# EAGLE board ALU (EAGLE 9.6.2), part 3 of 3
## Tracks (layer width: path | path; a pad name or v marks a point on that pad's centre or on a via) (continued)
N/IN/N2  (via drill 0.35) (continued)
  Top 0.152: IC70.9 99.06,26.09 99.32,26.35 v99.54,26.35 | IC63.10 127,41.28 v127.48,40.8
  Route3 0.152: v99.54,26.35 103.5,26.35 108.74,31.59 109.7,31.59 118.75,40.64 120.65,40.64 122.56,42.55 125.73,42.55 v127.48,40.8
  Bottom 0.152: 101.44,24.45 v99.54,26.35
N/IN/N3  (via drill 0.35)
  Top 0.152: v99.06,15.24 IC70.6 | v125.73,40.96 IC63.11
  Route3 0.152: v125.73,40.96 125.73,39.69 113.67,27.62 112.08,27.62 99.69,15.24 v99.06,15.24
STA  (via drill 0.35)
  Top 0.152: v109.22,46.99 IC67.13 | v139.7,47.47 IC56.13
  Route14 0.152: v139.7,47.47 139.38,47.15 114.14,47.15 113.19,46.2 110.01,46.2 v109.22,46.99
  Route15 0.152: v109.22,46.99 78.74,16.51 W.1
SUA  (via drill 0.35)
  Top 0.152: v113.03,40.64 IC66.10 | v115.41,56.2 111.44,56.2 110.49,57.15 IC68.12 | v139.7,67.31 IC58.13
  Route3 0.152: v139.7,67.31 135.57,63.18 122.4,63.18 v115.41,56.2 115.41,52.23 115.09,51.91 115.09,48.58 117,46.67 117,43.82 113.82,40.64 v113.03,40.64
SUB/IN/Z-/N0/0  (via drill 0.35)
  Top 0.152: v45.72,62.71 48.26,62.71 IC21.1 | v57.15,62.87 62.23,62.87 IC22.1 | v69.22,76.2 IC26.10
  Route2 0.152: v57.15,62.87 56.99,62.71 v45.72,62.71
  Route3 0.152: v69.22,76.2 65.88,72.87 65.88,70.96 65.41,70.48 63.5,70.48 57.15,64.14 v57.15,62.87
SUB/IN/Z-/N1/0
  Top 0.152: IC21.8 55.88,71.12 60.64,75.88 66.36,75.88 67.94,74.3 IC26.6 67.94,72.39 68.58,71.75 69.22,71.75 69.85,71.12 IC22.8
SUB/IN/Z-/N2/0  (via drill 0.35)
  Top 0.152: IC25.1 7.62,61.59 8.26,60.96 v8.89,60.96 | v64.14,74.93 64.77,74.93 65.41,74.3 IC26.4 | v19.37,62.71 19.37,62.87 19.47,62.97 IC24.1
  Route3 0.152: v64.14,74.93 57.78,68.58 35.56,68.58 34.77,69.37 32.54,69.37 31.27,70.64 29.53,70.64 21.59,62.71 v19.37,62.71
  Route14 0.152: v19.37,62.71 17.78,62.71 14.92,59.85 10,59.85 v8.89,60.96
SUB/IN/Z-/N3/0  (via drill 0.35)
  Top 0.152: IC25.8 15.24,70.48 16.51,71.75 26.67,71.75 27.94,70.48 27.94,69.22 | v59.69,73.66 60.96,74.93 62.55,74.93 62.87,74.61 IC26.2 | 27.94,69.22 v29.84,67.31 | 27.94,69.22 IC24.8
  Route2 0.152: v59.69,73.66 46.99,73.66 40.64,67.31 v29.84,67.31
SUB/OUT/N0  (via drill 0.35)
  Top 0.152: IC48.13 8.89,80.64 11.43,83.19 19.05,83.19 31.75,70.48 v31.75,66.04 | v31.75,51.44 32.38,50.8 36.2,50.8 36.83,51.44 IC18.3
  Bottom 0.152: v31.75,51.44 31.75,60.33 v31.75,66.04
SUB/OUT/N1  (via drill 0.35)
  Top 0.152: IC18.4 38.1,51.12 37.15,50.16 31.43,50.16 30.48,51.12 v30.48,54.61 | IC48.9 13.97,78.11 14.61,77.47 24.13,77.47 31.11,70.48 31.11,66.83 30.48,66.2 v30.48,64.77
  Bottom 0.152: v30.48,64.77 v30.48,54.61
SUB/OUT/N2  (via drill 0.35)
  Top 0.152: v29.53,69.37 29.53,70.8 25.4,74.93 14.61,74.93 13.97,74.3 IC48.6 | v36.83,60.64 39.05,60.64 39.37,60.33 IC18.10
  Route3 0.152: v29.53,69.37 36.83,62.07 v36.83,60.64
SUB/OUT/N3  (via drill 0.35)
  Top 0.152: v8.89,74.93 IC48.2 | IC18.11 v38.1,57.47
  Route15 0.152: v38.1,57.47 37.62,57.94 33.5,57.94 31.91,56.36 27.46,56.36 v8.89,74.93
SUB/OUT/Z-/N0  (via drill 0.35)
  Top 0.152: IC23.3 36.83,61.59 37.31,61.12 43.66,61.12 v48.26,56.52 49.53,55.25 IC16.2 | IC17.2 63.5,52.07 v62.23,50.8
  Route14 0.152: v48.26,56.52 48.58,56.2 54.61,56.2 58.98,51.83 61.2,51.83 v62.23,50.8
SUB/OUT/Z-/N1  (via drill 0.35)
  Top 0.152: IC23.4 38.1,61.91 38.42,61.59 46.67,61.59 v47.31,60.96 | v53.98,57.15 54.61,57.79 IC16.9 | v68.58,57.47 IC17.9
  Route2 0.152: v47.31,60.96 49.53,60.96 53.34,57.15 v53.98,57.15 54.45,57.63 63.34,57.63 65.09,55.88 66.99,55.88 v68.58,57.47
SUB/OUT/Z-/N2  (via drill 0.35)
  Top 0.152: IC19.2 21.59,54.61 20,56.2 17.46,56.2 16.35,55.09 9.68,55.09 v8.89,54.29 IC20.2 | IC23.10 39.37,71.12 37.47,73.03 v36.2,73.03
  Route2 0.152: v36.2,73.03 10.16,73.03 7.62,70.48 7.62,55.56 v8.89,54.29
SUB/OUT/Z-/N3  (via drill 0.35)
  Top 0.152: v19.05,57.15 14.61,57.15 13.97,57.79 IC20.9 | IC19.9 v26.67,60.33 28.57,60.33 32.23,63.98 32.23,65.27 33.68,66.72 33.68,70.25 35.67,72.23 37.62,72.23 38.1,71.75 IC23.11
  Route3 0.152: v19.05,57.15 19.21,57.31 23.02,57.31 26.04,60.33 v26.67,60.33
SUN  (via drill 0.35)
  Top 0.152: IC68.13 109.22,57.79 107.31,55.88 v107.31,55.25 | v109.86,33.02 110.49,32.38 IC66.3 | IC58.1 138.43,61.44 v131.13,54.13
  Route15 0.152: v131.13,54.13 129.38,52.39 121.92,52.39 120.97,53.34 109.22,53.34 v107.31,55.25
  Bottom 0.152: v107.31,55.25 107.31,35.56 v109.86,33.02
